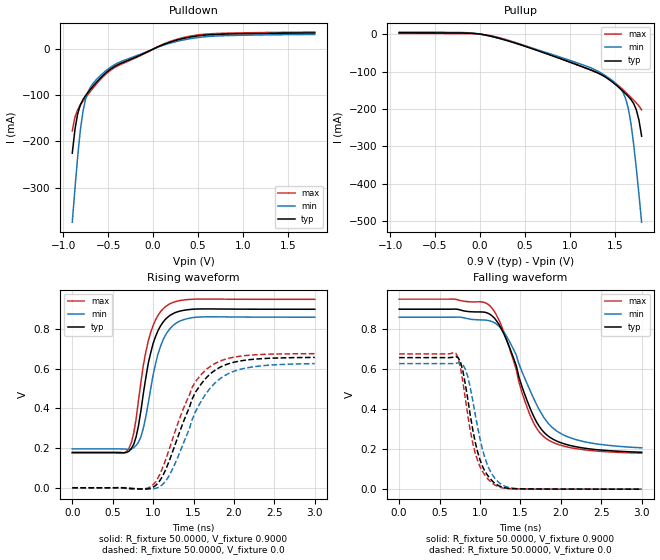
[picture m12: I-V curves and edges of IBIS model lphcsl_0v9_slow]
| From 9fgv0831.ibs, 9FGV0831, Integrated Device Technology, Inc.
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[Model]   lphcsl_0v9_slow
Model_type Output
Polarity   Non-Inverting
Enable   Active-High
Vmeas =  0.4000V
Cref =   2.0000pF
Rref =   0.0
Vref =   0.4000V
C_comp   1.1000pF   1.0000pF   1.2000pF
[Temperature Range]   25.0000   75.0000   0.0
[Voltage Range]   0.9000V   0.8600V   0.9500V
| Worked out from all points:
|   slope of the pulldown table from 0 to 0.135 V, typ, clamps not added: 11.8 ohm
|   slope of the pullup table from 0 to 0.135 V, typ, clamps not added: 21.1 ohm
|   rising waveform, R_fixture 50.0000, V_fixture 0.9000: 20-80 % time 201ps typ, 211ps min, 198ps max; typ from 0.178 V to 0.9 V
|   rising waveform, R_fixture 50.0000, V_fixture 0.0: 20-80 % time 404ps typ, 428ps min, 385ps max; typ from 0 V to 0.657 V
|   falling waveform, R_fixture 50.0000, V_fixture 0.9000: 20-80 % time 395ps typ, 452ps min, 374ps max; typ from 0.9 V to 0.185 V
|   falling waveform, R_fixture 50.0000, V_fixture 0.0: 20-80 % time 196ps typ, 206ps min, 192ps max; typ from 0.658 V to 0 V
[Pulldown]
|Voltage   I(typ)   I(min)   I(max)
-900mV    -225.6mA   -375.2mA   -177.4mA
-870mV    -174mA     -302.4mA   -147.5mA
-840mV    -140.3mA   -233.2mA   -131.2mA
-810mV    -120.8mA   -175.3mA   -121mA
-780mV    -109mA     -133.7mA   -112.8mA
-750mV    -100.2mA   -107mA     -105mA
-720mV    -92.49mA   -90.68mA   -97.27mA
-660mV    -78.35mA   -72.31mA   -82.41mA
-510mV    -48.82mA   -44.52mA   -51.32mA
90mV      7.972mA    6.753mA    8.709mA
390mV     25.27mA    21.84mA    27.29mA
1.8V      35.12mA    31.84mA    36.91mA
[Pullup]
|Voltage   I(typ)   I(min)   I(max)
-900mV    3.551mA    5.396mA    1.738mA
-150mV    2.686mA    3.793mA    1.334mA
150mV     -7.265mA   -7.528mA   -5.877mA
1.17V     -89.91mA   -84.27mA   -90.34mA
1.47V     -127.4mA   -123.7mA   -124.2mA
1.59V     -152mA     -154.4mA   -147.8mA
1.62V     -158.9mA   -170.8mA   -154.6mA
1.65V     -166.1mA   -197.2mA   -161.6mA
1.68V     -174.3mA   -237.1mA   -168.8mA
1.74V     -201.6mA   -356.7mA   -183.8mA
1.77V     -229.7mA   -428mA     -192mA
1.8V      -272.8mA   -502.6mA   -202.5mA
[Ramp]
| variable   typ   min   max
dV/dt_r  0.3943/0.4242n   0.3755/0.4479n   0.4056/0.4050n
dV/dt_f  0.4291/0.4154n   0.3919/0.4724n   0.4619/0.3943n
R_load = 50.0000
[Rising Waveform]
R_fixture= 50.0000
V_fixture= 0.9000
V_fixture_min= 0.8600
V_fixture_max= 0.9500
|time   V(typ)   V(min)   V(max)
0s        178.3mV    195.9mV    175.1mV
700ps     183.7mV    194mV      197.9mV
760ps     218.5mV    201.7mV    274.7mV
790ps     256.9mV    213.6mV    347.5mV
850ps     390.5mV    257.5mV    533.4mV
940ps     627.2mV    426.9mV    739.1mV
1.06ns    791.7mV    674.1mV    868.1mV
1.18ns    859.6mV    786.9mV    920.6mV
1.52ns    900.9mV    859.3mV    951mV
3ns       900mV      860.1mV    950mV
[Rising Waveform]
R_fixture= 50.0000
V_fixture= 0.0
V_fixture_min= 0.0
V_fixture_max= 0.0
|time   V(typ)   V(min)   V(max)
0s        0V         0V         0V
850ps     -6.349mV   -5.106mV   -6.787mV
1ns       2.978mV    -5.74mV    15.59mV
1.09ns    39.48mV    7.824mV    72.53mV
1.21ns    146.6mV    69.33mV    207.3mV
1.48ns    444.4mV    340.3mV    502.7mV
1.61ns    531.4mV    446.4mV    577.3mV
1.76ns    590.6mV    525.5mV    625.1mV
2.15ns    643.7mV    603.7mV    666.8mV
3ns       657.1mV    625.9mV    676mV
[Falling Waveform]
R_fixture= 50.0000
V_fixture= 0.9000
V_fixture_min= 0.8600
V_fixture_max= 0.9500
|time   V(typ)   V(min)   V(max)
0s        900mV      860mV      950mV
1.09ns    881.1mV    844.3mV    926.9mV
1.21ns    838.6mV    823.1mV    865.7mV
1.33ns    744.3mV    763.2mV    747mV
1.45ns    615.8mV    669.3mV    596.8mV
1.61ns    415mV      502.5mV    379.4mV
1.79ns    285.2mV    358.4mV    262mV
1.94ns    242.6mV    293.7mV    227.7mV
2.18ns    212.9mV    248.7mV    203.3mV
3ns       184.8mV    206.9mV    180.1mV
[Falling Waveform]
R_fixture= 50.0000
V_fixture= 0.0
V_fixture_min= 0.0
V_fixture_max= 0.0
|time   V(typ)   V(min)   V(max)
0s        657.8mV    627.8mV    676.3mV
700ps     663.3mV    629.2mV    680.1mV
760ps     634.5mV    631.4mV    605.7mV
820ps     522.5mV    599.6mV    449.8mV
880ps     369.4mV    507.4mV    292mV
940ps     237mV      377.5mV    181.1mV
1.06ns    90.28mV    158.1mV    70.74mV
1.18ns    30.74mV    56.34mV    22.02mV
1.48ns    1.603mV    2.538mV    1.331mV
3ns       117.1uV    175.9uV    92.31uV
